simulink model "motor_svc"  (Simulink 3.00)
settings: Solver=ode45  StartTime=0.0  StopTime=2.5  RelTol=1e-6  AbsTol=1e-6
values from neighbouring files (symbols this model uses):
  A = [-Ra Xq ; -Xdp -Ra]    [Gsinc.m]    (also in Cinic.m = -Xs*(Xm+Xr)-Xr*Xm; ptaylor.m = 0; Tdqf.m = [sin(u(3)) cos(u(3)); - cos(u(3)) sin(u(3))]; Tfdq.m = [sin(u(3)) cos(u(3)); - cos(u(3)) sin(u(3))])
  Ac = real(z(1,1))    [ptaylor.m]    (also in workspace_ctes.m = 0.0095)
  As = real(z(1,1))    [ptaylor.m]    (also in workspace_ctes.m = 0.035)
  B = [0 u(3)]'    [Gsinc.m]    (also in Cinic.m = Rs*(Xm+Xr); ptaylor.m = 0; workspace_ctes.m = 0)
  Bc = imag(z(1,1))    [ptaylor.m]    (also in workspace_ctes.m = 0.1279)
  Bs = imag(z(1,1))    [ptaylor.m]    (also in workspace_ctes.m = 0.2438)
  C = Pm*A^2+Pm*B^2-Rs*(Xm+Xr)^2    [Cinic.m]    (also in ptaylor.m = 0; workspace_ctes.m = 0)
  Cc = real(z(2,1))    [ptaylor.m]    (also in workspace_ctes.m = -0.3544)
  Cs = real(z(2,1))    [ptaylor.m]    (also in workspace_ctes.m = -0.678)
  D = 2*Pm*Rs*Rr*A+2*Pm*(Xs*Rr+Rr*Xm)*B-Rr*Xm^2    [Cinic.m]    (also in ptaylor.m = 0; workspace_ctes.m = 0)
  Dc = imag(z(2,1))    [ptaylor.m]    (also in workspace_ctes.m = 0.0093)
  Ds = imag(z(2,1))    [ptaylor.m]    (also in workspace_ctes.m = 0.0644)
  Imv = Imv'    [ptaylor.m]    (also in workspace_ctes.m = [-0.0879 -1.7628 -0.2794 1.4912])
  Imvc = Imvc'    [ptaylor.m]    (also in workspace_ctes.m = [-0.0175 -0.6693 -0.2556 1.8032])
  Imvs = Imvs'    [ptaylor.m]    (also in workspace_ctes.m = [-0.1217 -1.2805 -0.3651 0.9022])
  U3v = U3v'    [ptaylor.m]    (also in workspace_ctes.m = [0.6354 -0.0622 0.4667 -0.0233])
  U3vc = U3vc'    [ptaylor.m]    (also in workspace_ctes.m = [0.2415 -0.0179 0.3544 -0.0093])
  U3vs = U3vs'    [ptaylor.m]    (also in workspace_ctes.m = [0.4605 -0.0661 0.6780 -0.0644])

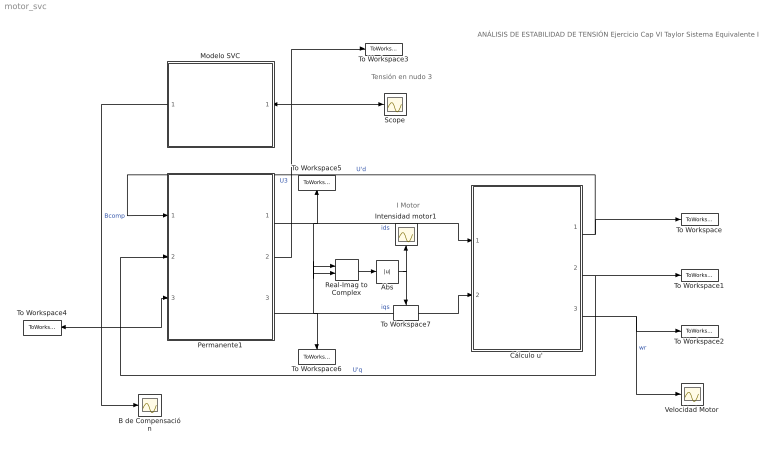
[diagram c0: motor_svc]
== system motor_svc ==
  note: ANÁLISIS DE ESTABILIDAD DE TENSIÓN Ejercicio Cap VI Taylor Sistema Equivalente I
  note: Tensión en nudo 3
  note: I Motor
  Abs : Abs
  B de Compensación : Scope
  Cálculo u' : Subsystem  mask(Modelo del rotor  del motor){Um=1, Pm=0.6, Am=1, Bm=0, Cm=0, Dm=0, Hm=0.7, Xm=3.2, Xr=0.18, Rr=0.018, Xs=0.1, Rs=0.031}
      mask prompts: Um "Tensión de alimentación (p.u)"; Pm "Potencia en el eje (p.u.)"; Am "Parámetro A modelo de Tcarga"; Bm "Parámetro B modelo de Tcarga"; Cm "Parámetro C modelo de Tcarga"; Dm "Parámetro D modelo de Tcarga"; Hm "Inercia,  H (s)"; Xm "Reactancia de Magnetización,  Xm (p.u.)"; Xr "Reactancia Rotor,  Xr  (p.u.)"; Rr "Resistencia del Rotor,  Rr  (p.u.)"; Xs "Reactancia del estator,  Xs  (p.u.)"; Rs "Resistencia del estator,  Rs  (p.u.)"
  Intensidad motor1 : Scope
  Modelo SVC : Subsystem  Orientation=left  mask{Tc=0, Bmin=-0.15, Bmax=0.25, Ta=0.05, G=50}
      mask prompts: Tc "Instante Entrada SVC (s)"; Bmin "Bmin (p.u.)"; Bmax "Bmax  (p.u.)"; Ta "Cte. Tiempo SVC (s)"; G "Ganancia"
  Permanente1 : Subsystem
  Real-Imag to Complex : RealImagToComplex  Input=RealAndImag  ConstantPart=0
  Scope : Scope
  To Workspace : ToWorkspace  VariableName=ud  SampleTime=0  SaveFormat=Matrix
  To Workspace1 : ToWorkspace  VariableName=uq  SampleTime=0  SaveFormat=Matrix
  To Workspace2 : ToWorkspace  VariableName=wr  SampleTime=0  SaveFormat=Matrix
  To Workspace3 : ToWorkspace  VariableName=U3  SampleTime=0  SaveFormat=Matrix
  To Workspace4 : ToWorkspace  VariableName=Bcomp  SampleTime=0  SaveFormat=Matrix
  To Workspace5 : ToWorkspace  VariableName=ids  SampleTime=0  SaveFormat=Matrix
  To Workspace6 : ToWorkspace  VariableName=iqs  SampleTime=0  SaveFormat=Matrix
  To Workspace7 : ToWorkspace  VariableName=Im  SampleTime=-1  SaveFormat=Matrix
  Velocidad Motor : Scope
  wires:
  Cálculo u'/2(u'q) -> To Workspace1/1, Permanente1/2(U'q)  "U'q"
  Cálculo u'/3(wr) -> To Workspace2/1, Velocidad Motor/1  "wr"
  Cálculo u'/1(u'd) -> To Workspace/1, Permanente1/1(U'd)  "U'd"
  Modelo SVC/1(Bcomp) -> Permanente1/3(B comp), B de Compensación/1, To Workspace4/1  "Bcomp"
  Permanente1/2(U3) -> Scope/1, To Workspace3/1, Modelo SVC/1(U3)  "U3"
  Permanente1/1(Im real) -> Cálculo u'/1(ids), To Workspace5/1, Real-Imag to Complex/1  "ids"
  Permanente1/3(Im imag) -> Cálculo u'/2(iqs), To Workspace6/1, Real-Imag to Complex/2  "iqs"
  Real-Imag to Complex/1 -> Abs/1
  Abs/1 -> To Workspace7/1, Intensidad motor1/1

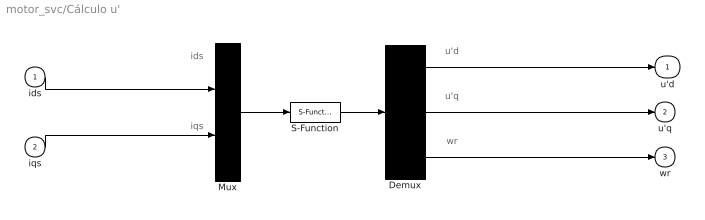
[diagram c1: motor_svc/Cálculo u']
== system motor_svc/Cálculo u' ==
  note: wr
  note: u'q
  note: u'd
  note: iqs
  note: ids
  ids : Inport  Port=1  PortWidth=-1  SampleTime=-1  DataType=auto
  iqs : Inport  Port=2  PortWidth=-1  SampleTime=-1  DataType=auto
  Demux : Demux  Outputs=3
  Mux : Mux  Inputs=2
  S-Function : S-Function  FunctionName=rotorind  Parameters=Rs, Xs, Rr, Xr, Xm, Hm, Am, Bm, Cm, Dm, Pm, Um  PortCounts=[]  SFunctionModules=''
  u'd : Outport  Port=1
  u'q : Outport  Port=2
  wr : Outport  Port=3
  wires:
  ids/1 -> Mux/1
  iqs/1 -> Mux/2
  S-Function/1 -> Demux/1
  Mux/1 -> S-Function/1
  Demux/1 -> u'd/1
  Demux/2 -> u'q/1
  Demux/3 -> wr/1

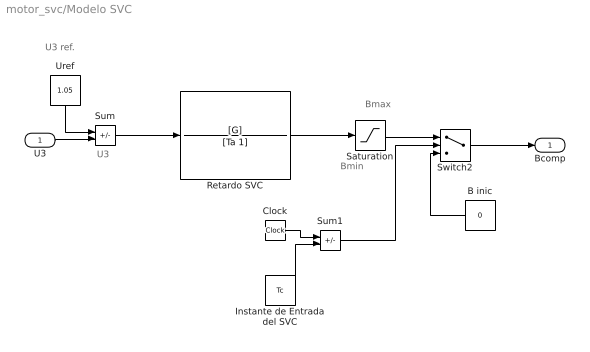
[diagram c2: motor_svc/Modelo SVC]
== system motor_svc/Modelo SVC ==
  note: U3
  note: Bmin
  note: Bmax
  note: U3 ref.
  U3 : Inport  Port=1  PortWidth=-1  SampleTime=-1  DataType=auto
  B inic : Constant  Orientation=left  Value=0
  Clock : Clock
  Instante de Entrada del SVC : Constant  Value=Tc
  Retardo SVC : TransferFcn  Numerator=[G]  Denominator=[Ta 1]
  Saturation : Saturate  UpperLimit=Bmax  LowerLimit=Bmin
  Sum : Sum  Inputs=+-  SaturateOnIntegerOverflow=on
  Sum1 : Sum  Inputs=+-  SaturateOnIntegerOverflow=on
  Switch2 : Switch  Threshold=0
  Uref : Constant  Orientation=down  Value=1.05
  Bcomp : Outport  Port=1
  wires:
  Retardo SVC/1 -> Saturation/1
  Uref/1 -> Sum/1
  Sum/1 -> Retardo SVC/1
  Saturation/1 -> Switch2/1
  B inic/1 -> Switch2/3
  Clock/1 -> Sum1/1
  Instante de Entrada del SVC/1 -> Sum1/2
  Sum1/1 -> Switch2/2
  U3/1 -> Sum/2
  Switch2/1 -> Bcomp/1

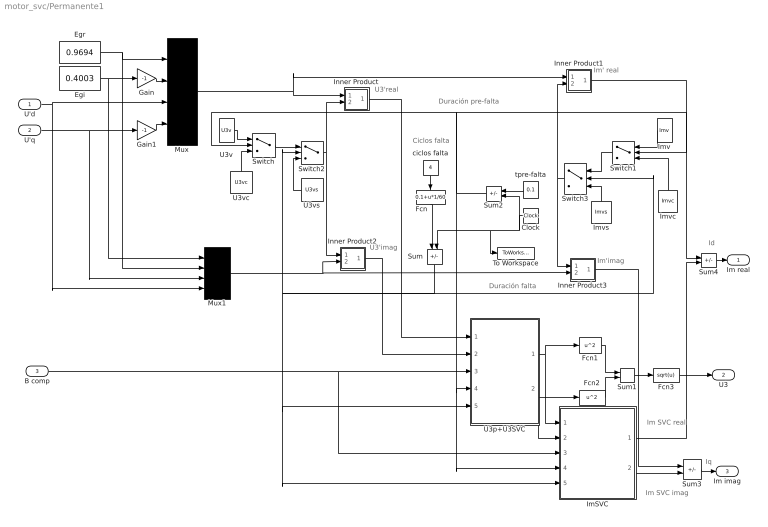
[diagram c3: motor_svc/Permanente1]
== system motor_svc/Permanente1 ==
  note: Im SVC imag
  note: Im SVC real
  note: Duración falta
  note: Duración pre-falta
  note: Ciclos falta
  note: Iq
  note: Id
  note: Im'imag
  note: Im' real
  note: U3'imag
  note: U3'real
  U'd : Inport  Port=1  PortWidth=-1  SampleTime=-1  DataType=auto
  U'q : Inport  Port=2  PortWidth=-1  SampleTime=-1  DataType=auto
  B comp : Inport  Port=3  PortWidth=-1  SampleTime=-1  DataType=auto
  Clock : Clock
  Egi : Constant  Value=0.4003
  Egr : Constant  Value=0.9694
  Fcn : Fcn  Orientation=down  Expr=0.1+u*1/60
  Fcn1 : Fcn  Expr=u^2
  Fcn2 : Fcn  Expr=u^2
  Fcn3 : Fcn  Expr=sqrt(u)
  Gain : Gain  Gain=-1  SaturateOnIntegerOverflow=on
  Gain1 : Gain  Gain=-1  SaturateOnIntegerOverflow=on
  ImSVC : Subsystem
  Imv : Constant  Orientation=left  Value=Imv
  Imvc : Constant  Orientation=up  Value=Imvc
  Imvs : Constant  Orientation=up  Value=Imvs
  Inner Product : Subsystem
  Inner Product1 : Subsystem
  Inner Product2 : Subsystem
  Inner Product3 : Subsystem
  Mux : Mux  Inputs=4
  Mux1 : Mux  Inputs=4
  Sum : Sum  Orientation=down  Inputs=+-  SaturateOnIntegerOverflow=on
  Sum1 : Sum  Inputs=++  SaturateOnIntegerOverflow=on
  Sum2 : Sum  Orientation=left  Inputs=+-  SaturateOnIntegerOverflow=on
  Sum3 : Sum  Inputs=+-  SaturateOnIntegerOverflow=on
  Sum4 : Sum  Inputs=+-  SaturateOnIntegerOverflow=on
  Switch : Switch  Threshold=0
  Switch1 : Switch  Orientation=left  Threshold=0
  Switch2 : Switch  Threshold=0
  Switch3 : Switch  Orientation=left  Threshold=0
  To Workspace : ToWorkspace  VariableName=t  SampleTime=0  SaveFormat=Matrix
  U3p+U3SVC : Subsystem
  U3v : Constant  Value=U3v
  U3vc : Constant  Orientation=up  Value=U3vc
  U3vs : Constant  Orientation=left  Value=U3vs
  ciclos falta : Constant  Orientation=down  Value=4
  tpre-falta : Constant  Orientation=left  Value=0.1
  Im real : Outport  Port=1
  U3 : Outport  Port=2
  Im imag : Outport  Port=3
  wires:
  Inner Product1/1(out_1) -> Sum4/1
  U3v/1 -> Switch/1
  Switch2/1 -> Inner Product/2(in_2), Inner Product2/1(in_1)
  ciclos falta/1 -> Fcn/1
  Fcn/1 -> Sum/1
  Mux/1 -> Inner Product/1(in_1), Inner Product1/1(in_1)
  Inner Product/1(out_1) -> U3p+U3SVC/1(U3' real)
  U3vs/1 -> Switch2/3
  Switch/1 -> Switch2/1
  U3vc/1 -> Switch/3
  Sum2/1 -> ImSVC/4(T pre-falta), U3p+U3SVC/4(T pre-falta), Switch/2, Switch1/2
  Clock/1 -> To Workspace/1, Sum/2, Sum2/2
  tpre-falta/1 -> Sum2/1
  Sum/1 -> ImSVC/5(T falta), U3p+U3SVC/5(T falta), Switch3/2, Switch2/2
  Imvs/1 -> Switch3/3
  Switch1/1 -> Switch3/1
  Switch3/1 -> Inner Product1/2(in_2), Inner Product3/1(in_1)
  Imv/1 -> Switch1/1
  Imvc/1 -> Switch1/3
  Gain1/1 -> Mux/4
  Sum3/1 -> Im imag/1
  Fcn3/1 -> U3/1
  Sum4/1 -> Im real/1
  Mux1/1 -> Inner Product2/2(in_2), Inner Product3/2(in_2)
  U'd/1 -> Mux1/4, Mux/3
  U'q/1 -> Mux1/3, Gain1/1
  Egr/1 -> Mux1/2, Mux/1
  Egi/1 -> Mux1/1, Gain/1
  Gain/1 -> Mux/2
  ImSVC/1("Im SVC real ") -> Sum4/2
  Inner Product3/1(out_1) -> Sum3/1
  ImSVC/2("Im SVC imag ") -> Sum3/2
  B comp/1 -> ImSVC/3(Bcomp), U3p+U3SVC/3(Bcomp)
  U3p+U3SVC/2(U3 imag) -> ImSVC/2(U3imag), Fcn2/1
  U3p+U3SVC/1(U3 real) -> ImSVC/1(U3 real), Fcn1/1
  Sum1/1 -> Fcn3/1
  Fcn2/1 -> Sum1/2
  Fcn1/1 -> Sum1/1
  Inner Product2/1(out_1) -> U3p+U3SVC/2(U3'imag)

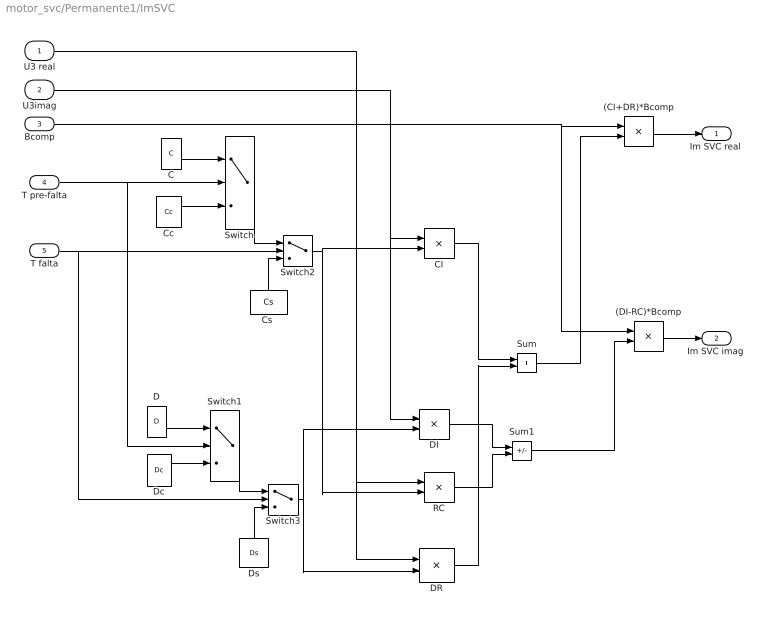
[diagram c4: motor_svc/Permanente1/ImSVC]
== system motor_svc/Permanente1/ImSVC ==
  U3 real : Inport  Port=1  PortWidth=-1  SampleTime=-1  DataType=auto
  U3imag : Inport  Port=2  PortWidth=-1  SampleTime=-1  DataType=auto
  Bcomp : Inport  Port=3  PortWidth=-1  SampleTime=-1  DataType=auto
  T pre-falta : Inport  Port=4  PortWidth=-1  SampleTime=-1  DataType=auto
  T falta : Inport  Port=5  PortWidth=-1  SampleTime=-1  DataType=auto
  (CI+DR)*Bcomp : Product  Inputs=2  SaturateOnIntegerOverflow=on
  (DI-RC)*Bcomp : Product  Inputs=2  SaturateOnIntegerOverflow=on
  C : Constant  Value=C
  CI : Product  Inputs=2  SaturateOnIntegerOverflow=on
  Cc : Constant  Value=Cc
  "Cs " : Constant  Orientation=up  Value=Cs
  D : Constant  Value=D
  DI : Product  Inputs=2  SaturateOnIntegerOverflow=on
  DR : Product  Inputs=2  SaturateOnIntegerOverflow=on
  Dc : Constant  Value=Dc
  Ds : Constant  Orientation=up  Value=Ds
  RC : Product  Inputs=2  SaturateOnIntegerOverflow=on
  Sum : Sum  Inputs=++  SaturateOnIntegerOverflow=on
  Sum1 : Sum  Inputs=+-  SaturateOnIntegerOverflow=on
  Switch{,1..3} (4 alike) : Switch  Threshold=0
  "Im SVC real " : Outport  Port=1
  "Im SVC imag " : Outport  Port=2
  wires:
  Switch3/1 -> DI/2, DR/2
  D/1 -> Switch1/1
  Dc/1 -> Switch1/3
  Ds/1 -> Switch3/3
  Switch1/1 -> Switch3/1
  (DI-RC)*Bcomp/1 -> "Im SVC imag "/1
  (CI+DR)*Bcomp/1 -> "Im SVC real "/1
  Bcomp/1 -> (DI-RC)*Bcomp/1, (CI+DR)*Bcomp/1
  Sum1/1 -> (DI-RC)*Bcomp/2
  RC/1 -> Sum1/2
  DI/1 -> Sum1/1
  Switch2/1 -> RC/2, CI/2
  U3 real/1 -> RC/1, DR/1
  U3imag/1 -> DI/1, CI/1
  Sum/1 -> (CI+DR)*Bcomp/2
  DR/1 -> Sum/2
  CI/1 -> Sum/1
  T falta/1 -> Switch3/2, Switch2/2
  T pre-falta/1 -> Switch1/2, Switch/2
  C/1 -> Switch/1
  Cc/1 -> Switch/3
  "Cs "/1 -> Switch2/3
  Switch/1 -> Switch2/1

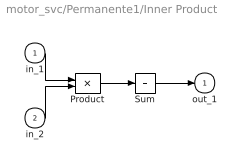
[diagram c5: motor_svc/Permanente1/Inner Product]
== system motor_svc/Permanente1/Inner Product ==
  in_1 : Inport  Port=1  PortWidth=-1  SampleTime=-1  DataType=auto
  in_2 : Inport  Port=2  PortWidth=-1  SampleTime=-1  DataType=auto
  Product : Product  Inputs=2  SaturateOnIntegerOverflow=on
  Sum : Sum  Inputs=+  SaturateOnIntegerOverflow=on
  out_1 : Outport  Port=1
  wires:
  Sum/1 -> out_1/1
  Product/1 -> Sum/1
  in_1/1 -> Product/1
  in_2/1 -> Product/2

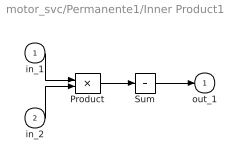
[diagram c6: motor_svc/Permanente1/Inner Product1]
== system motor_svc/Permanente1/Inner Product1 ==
  in_1 : Inport  Port=1  PortWidth=-1  SampleTime=-1  DataType=auto
  in_2 : Inport  Port=2  PortWidth=-1  SampleTime=-1  DataType=auto
  Product : Product  Inputs=2  SaturateOnIntegerOverflow=on
  Sum : Sum  Inputs=+  SaturateOnIntegerOverflow=on
  out_1 : Outport  Port=1
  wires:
  Sum/1 -> out_1/1
  Product/1 -> Sum/1
  in_1/1 -> Product/1
  in_2/1 -> Product/2

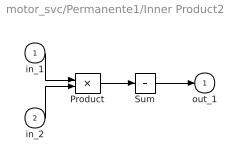
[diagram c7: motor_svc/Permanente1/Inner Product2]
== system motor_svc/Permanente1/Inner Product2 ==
  in_1 : Inport  Port=1  PortWidth=-1  SampleTime=-1  DataType=auto
  in_2 : Inport  Port=2  PortWidth=-1  SampleTime=-1  DataType=auto
  Product : Product  Inputs=2  SaturateOnIntegerOverflow=on
  Sum : Sum  Inputs=+  SaturateOnIntegerOverflow=on
  out_1 : Outport  Port=1
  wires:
  Sum/1 -> out_1/1
  Product/1 -> Sum/1
  in_1/1 -> Product/1
  in_2/1 -> Product/2

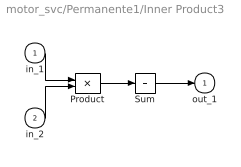
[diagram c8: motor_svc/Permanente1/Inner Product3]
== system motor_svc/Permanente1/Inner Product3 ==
  in_1 : Inport  Port=1  PortWidth=-1  SampleTime=-1  DataType=auto
  in_2 : Inport  Port=2  PortWidth=-1  SampleTime=-1  DataType=auto
  Product : Product  Inputs=2  SaturateOnIntegerOverflow=on
  Sum : Sum  Inputs=+  SaturateOnIntegerOverflow=on
  out_1 : Outport  Port=1
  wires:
  Sum/1 -> out_1/1
  Product/1 -> Sum/1
  in_1/1 -> Product/1
  in_2/1 -> Product/2

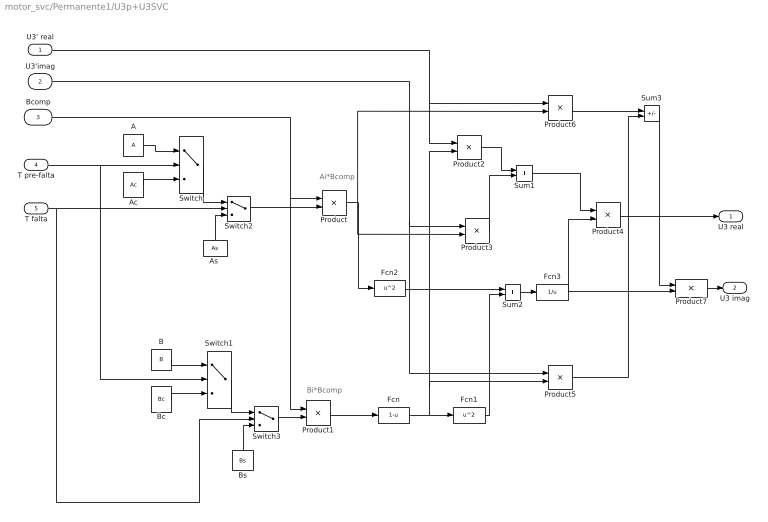
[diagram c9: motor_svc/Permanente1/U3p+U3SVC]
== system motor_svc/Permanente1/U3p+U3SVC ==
  note: Ai*Bcomp
  note: Bi*Bcomp
  U3' real : Inport  Port=1  PortWidth=-1  SampleTime=-1  DataType=auto
  U3'imag : Inport  Port=2  PortWidth=-1  SampleTime=-1  DataType=auto
  Bcomp : Inport  Port=3  PortWidth=-1  SampleTime=-1  DataType=auto
  T pre-falta : Inport  Port=4  PortWidth=-1  SampleTime=-1  DataType=auto
  T falta : Inport  Port=5  PortWidth=-1  SampleTime=-1  DataType=auto
  A : Constant  Value=A
  Ac : Constant  Value=Ac
  "As " : Constant  Orientation=up  Value=As
  B : Constant  Value=B
  Bc : Constant  Value=Bc
  Bs : Constant  Orientation=up  Value=Bs
  Fcn : Fcn  Expr=1-u
  Fcn1 : Fcn  Expr=u^2
  Fcn2 : Fcn  Expr=u^2
  Fcn3 : Fcn  Expr=1/u
  Product{,1..7} (8 alike) : Product  Inputs=2  SaturateOnIntegerOverflow=on
  Sum1 : Sum  Inputs=++  SaturateOnIntegerOverflow=on
  Sum2 : Sum  Inputs=++  SaturateOnIntegerOverflow=on
  Sum3 : Sum  Inputs=-+  SaturateOnIntegerOverflow=on
  Switch{,1..3} (4 alike) : Switch  Threshold=0
  U3 real : Outport  Port=1
  U3 imag : Outport  Port=2
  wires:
  U3' real/1 -> Product6/1, Product2/1
  Bcomp/1 -> Product/1, Product1/1
  Product7/1 -> U3 imag/1
  Product4/1 -> U3 real/1
  Sum3/1 -> Product7/1
  Fcn3/1 -> Product7/2, Product4/2
  Product5/1 -> Sum3/2
  Product6/1 -> Sum3/1
  U3'imag/1 -> Product5/1, Product3/1
  Sum2/1 -> Fcn3/1
  Fcn1/1 -> Sum2/2
  Fcn2/1 -> Sum2/1
  Sum1/1 -> Product4/1
  Product/1 -> Product6/2, Product3/2, Fcn2/1
  Fcn/1 -> Product5/2, Product2/2, Fcn1/1
  Product1/1 -> Fcn/1
  Switch3/1 -> Product1/2
  Switch2/1 -> Product/2
  Product3/1 -> Sum1/2
  Product2/1 -> Sum1/1
  T falta/1 -> Switch3/2, Switch2/2
  T pre-falta/1 -> Switch1/2, Switch/2
  A/1 -> Switch/1
  Ac/1 -> Switch/3
  "As "/1 -> Switch2/3
  Switch/1 -> Switch2/1
  B/1 -> Switch1/1
  Bc/1 -> Switch1/3
  Bs/1 -> Switch3/3
  Switch1/1 -> Switch3/1
